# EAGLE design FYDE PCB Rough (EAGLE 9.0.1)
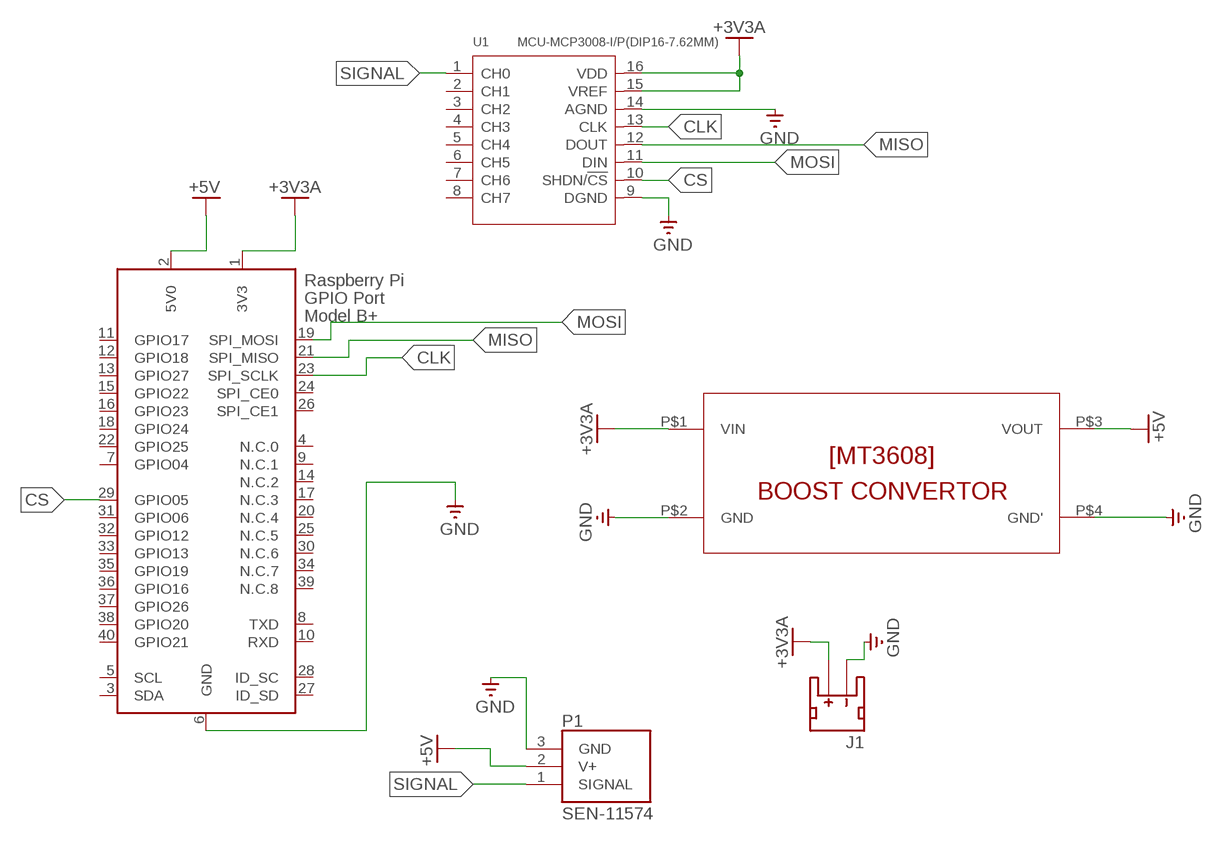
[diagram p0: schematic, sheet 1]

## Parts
J1  JST_2MM_MALE  [JST-2-SMD]
P1  SEN-11574  [XDCR_SEN-11574]
U1  MCU-MCP3008-I/P(DIP16-7.62MM)  [DIP16-2.54-19.2X7.62MM]
U$2  MT3608  [MT3608]
X1  RASPI_BOARD_B+_HDC  [RASPI_BOARD_B+HAT_DF_CF]

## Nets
+3V3A: J1.2(+) U1.15(VREF) U1.16(VDD) U$2.P$1(VIN) X1.1(3V3)
+5V: P1.2(V+) U$2.P$3(VOUT) X1.2(5V0)
CLK: U1.13(CLK) X1.23(SPI_SCLK)
CS: U1.10(SHDN/!CS) X1.29(GPIO05)
GND: J1.1(-) P1.3(GND) U1.9(DGND) U1.14(AGND) U$2.P$2(GND) U$2.P$4(GND') X1.6(GND)
MISO: U1.12(DOUT) X1.21(SPI_MISO)
MOSI: U1.11(DIN) X1.19(SPI_MOSI)
SIGNAL: P1.1(SIGNAL) U1.1(CH0)
Unconnected: J1.NC1(PAD1) J1.NC2(PAD2) U1.2(CH1) U1.3(CH2) U1.4(CH3) U1.5(CH4) U1.6(CH5) U1.7(CH6) U1.8(CH7) X1.3(SDA) X1.4(N.C.0) X1.5(SCL) X1.7(GPIO04) X1.8(TXD) X1.9(N.C.1) X1.10(RXD) X1.11(GPIO17) X1.12(GPIO18) X1.13(GPIO27) X1.14(N.C.2) X1.15(GPIO22) X1.16(GPIO23) X1.17(N.C.3) X1.18(GPIO24) X1.20(N.C.4) X1.22(GPIO25) X1.24(SPI_CE0) X1.25(N.C.5) X1.26(SPI_CE1) X1.27(ID_SD) X1.28(ID_SC) X1.30(N.C.6) X1.31(GPIO06) X1.32(GPIO12) X1.33(GPIO13) X1.34(N.C.7) X1.35(GPIO19) X1.36(GPIO16) X1.37(GPIO26) X1.38(GPIO20) X1.39(N.C.8) X1.40(GPIO21)

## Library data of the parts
J1 = SparkFun-Connectors:JST_2MM_MALE: JST 2MM MALE RA CONNECTOR Two pin, compact surface mount connector. Commonly used as a battery input connection point. We really like the solid locking feeling and high current rating on these small connectors. We use these all the time as battery connectors. Mates to single-cell LiPo batteries.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; PROD_ID: CONN-11443; SF_ID: PRT-08612
P1 = SEN-11574:SEN-11574: Pulse Sensor For Arduino; AVAILABILITY: Unavailable; DESCRIPTION: PULSE SENSOR FOR ARDUINO; MF: SparkFun; MP: SEN-11574; PACKAGE: None; PRICE: None
U1 = MCU-MCP3008-I_P_DIP16-7.62MM_:MCU-MCP3008-I/P(DIP16-7.62MM): 310990040; AVAILABILITY: Unavailable; DESCRIPTION: 10 Bit Analog to Digital Converter 4, 8 Input 1 SAR 16-PDIP; MF: Microchip; MP: MCP3008-I/P; PACKAGE: DIP-16 Microchip; PRICE: None
U$2 = MT3608:MT3608
X1 = raspberrypi_bastelstube_v13:RASPI_BOARD_B+: Raspberry Pi GPIO connector with markings for the outer dimensions of the Raspberry Pi board model B+ with different sets of drill holes or mounting pads

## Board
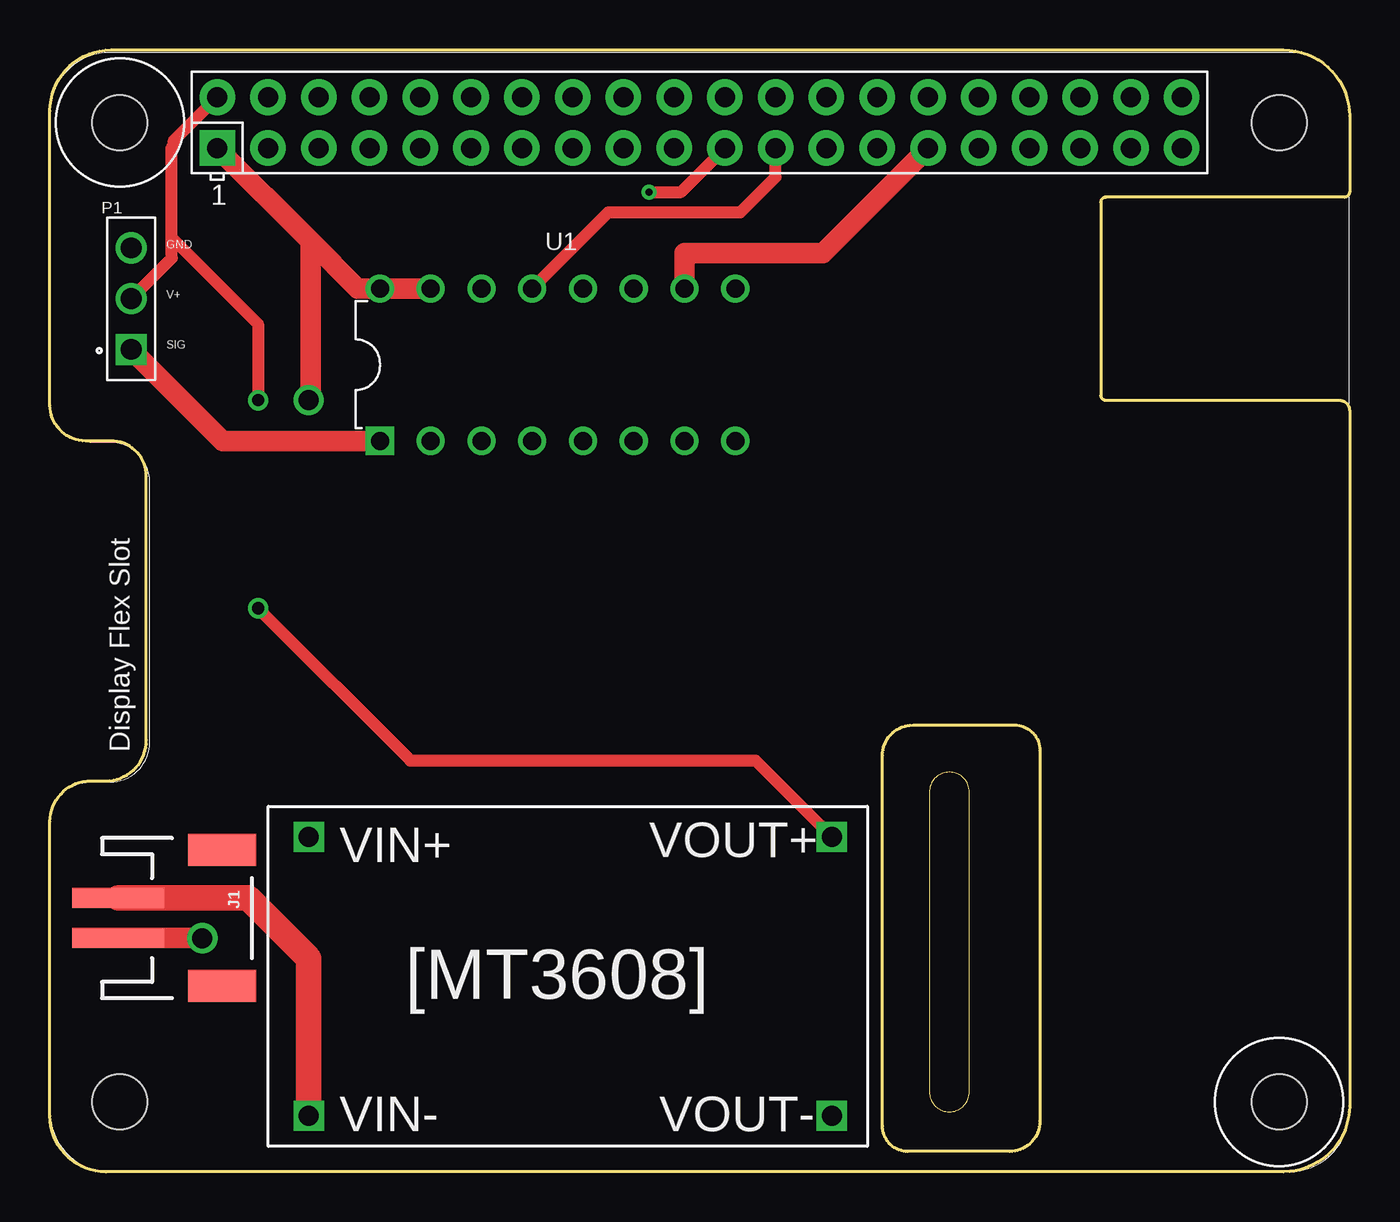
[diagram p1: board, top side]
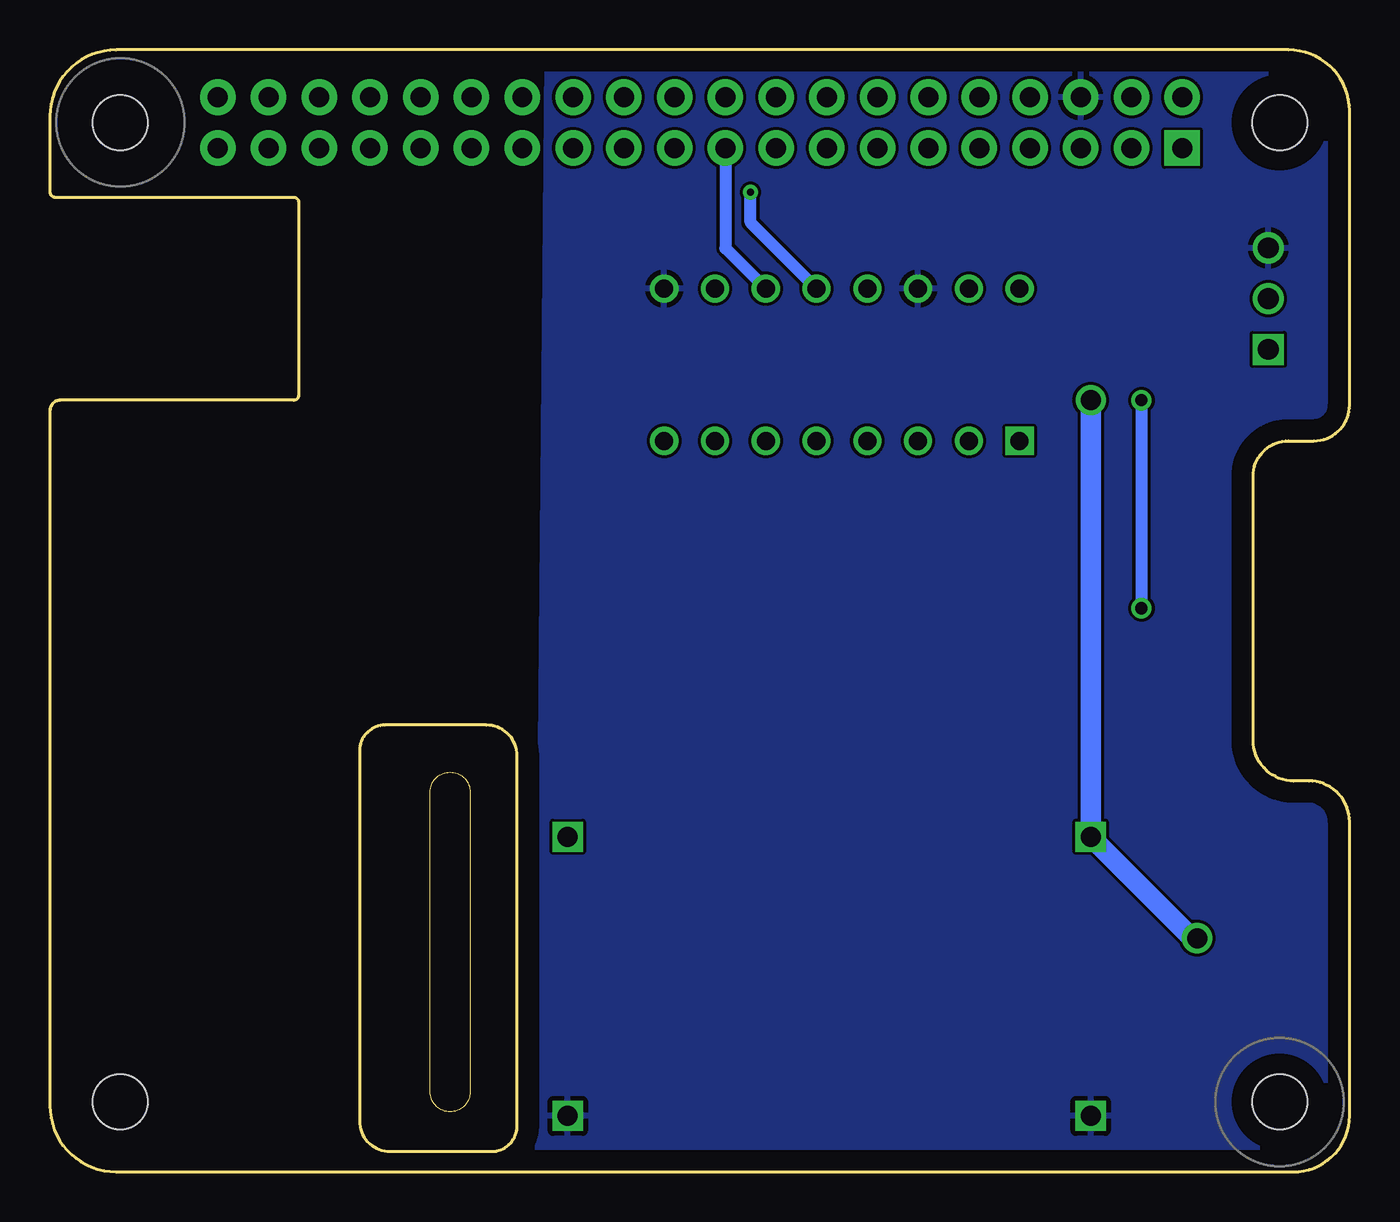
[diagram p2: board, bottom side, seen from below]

Size 65.02 x 56.13 mm. Coordinates in mm from the lower left corner, seen from the top.
Outline: 0,53.09 arc-90 3.05,56.13 61.72,56.13 arc-90 65.02,52.83 65.02,49.02 arc-90 64.77,48.77 52.83,48.77 arc90 52.58,48.51 52.58,38.86 arc90 52.83,38.61 64.52,38.61 arc-90 65.02,38.1 65.02,3.3 arc-90 61.72,0 2.79,0 arc-90 0,2.79 0,17.53 arc-90 2.03,19.56 2.79,19.56 arc90 4.83,21.59 4.83,34.8 arc90 3.05,36.58 1.78,36.58 arc-90 0,38.35 0,53.09
Outline: 41.66,2.29 41.66,20.83 arc-90 43.18,22.35 48.26,22.35 arc-90 49.53,21.08 49.53,2.54 arc-90 48.01,1.02 42.93,1.02 arc-90 41.66,2.29
Copper layers (1*16): Top 0.035mm / dielectric 1.5mm / Bottom 0.035mm
Design rules "default": minimum track width 6mil, minimum drill 0.35mm, track to track 6mil, track to pad 6mil, pad to pad 6mil, via to via 6mil, smd to smd 6mil, copper to edge 40mil, drill to drill 6mil, minimum pad ring 10mil, minimum via ring 8mil, stop-mask expansion 4mil, vias tented up to drill 0mil, thermal gap 10mil

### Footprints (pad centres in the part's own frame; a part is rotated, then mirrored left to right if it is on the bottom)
JST-2-SMD = smd 1 x 4.6: 1 -1,-3.7; 2 1,-3.7 | smd 1.6 x 3.4: NC1 -3.4,1.5; NC2 3.4,1.5
XDCR_SEN-11574 = drill 1.04 square: 1 0,-2.54 | drill 1.04: 2 0,0; 3 0,2.54
DIP16-2.54-19.2X7.62MM = drill 0.9 pad 1.4 square: 1 -8.89,-3.81 | drill 0.9 pad 1.4: 2 -6.35,-3.81; 3 -3.81,-3.81; 4 -1.27,-3.81; 5 1.27,-3.81; 6 3.81,-3.81; 7 6.35,-3.81; 8 8.89,-3.81; 9 8.89,3.81; 10 6.35,3.81; 11 3.81,3.81; 12 1.27,3.81; 13 -1.27,3.81; 14 -3.81,3.81; 15 -6.35,3.81; 16 -8.89,3.81
MT3608 = drill 1 square: P$1 2.032,15.494; P$2 2.032,1.524; P$3 28.194,15.494; P$4 28.194,1.524
RASPI_BOARD_B+HAT_DF_CF = drill 1 pad 1.778 square: 1 8.37,51.23 | drill 1 pad 1.778: 2 8.37,53.77; 3 10.91,51.23; 4 10.91,53.77; 5 13.45,51.23; 6 13.45,53.77; 7 15.99,51.23; 8 15.99,53.77; 9 18.53,51.23; 10 18.53,53.77; 11 21.07,51.23; 12 21.07,53.77; 13 23.61,51.23; 14 23.61,53.77; 15 26.15,51.23; 16 26.15,53.77; 17 28.69,51.23; 18 28.69,53.77; 19 31.23,51.23; 20 31.23,53.77; 21 33.77,51.23; 22 33.77,53.77; 23 36.31,51.23; 24 36.31,53.77; 25 38.85,51.23; 26 38.85,53.77; 27 41.39,51.23; 28 41.39,53.77; 29 43.93,51.23; 30 43.93,53.77; 31 46.47,51.23; 32 46.47,53.77; 33 49.01,51.23; 34 49.01,53.77; 35 51.55,51.23; 36 51.55,53.77; 37 54.09,51.23; 38 54.09,53.77; 39 56.63,51.23; 40 56.63,53.77 | hole 2.75: 3.5,3.5; 3.5,52.5; 61.5,3.5; 61.5,52.5

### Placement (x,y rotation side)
J1  7.11,12.7 270 top
P1  4.06,43.69 0 top
U1  25.4,40.39 0 top
U$2  10.92,1.27 0 top
X1  0,0 0 top

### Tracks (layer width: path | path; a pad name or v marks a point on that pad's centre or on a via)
+3V3A  (via drill 1, 1.02)
  Top 1.016: X1.1 13.04,46.56 | 13.04,46.56 15.4,44.2 U1.16 U1.15 | 13.04,46.56 13.04,38.69 v12.95,38.61 | J1.2 7.6,11.7 v7.62,11.68
  Bottom 1.016: v12.95,38.61 U$2.P$1 7.87,11.68 v7.62,11.68
+5V  (via drill 0.61)
  Top 0.61: P1.2 6.1,45.72 6.1,46.74 | X1.2 6.2,51.6 6.2,51.38 6.1,51.28 6.1,46.74 | 6.1,46.74 10.41,42.42 v10.41,38.61 | v10.41,28.19 18.03,20.57 32.26,20.57 35.31,20.57 U$2.P$3
  Bottom 0.61: v10.41,38.61 v10.41,28.19
CLK
  Top 0.61: U1.13 27.94,48.01 34.54,48.01 36.31,49.77 X1.23
CS
  Top 1.016: X1.29 38.67,45.97 31.75,45.97 U1.10
GND
  Top 1.27: J1.1 9.92,13.7 12.95,10.67 U$2.P$2
  pour Bottom: 0.51,55.63 1.02,0 40.64,0 40.13,55.63
MISO  (via drill 0.35)
  Top 0.61: v29.97,49.02 31.56,49.02 X1.21
  Bottom 0.61: U1.12 29.97,47.5 v29.97,49.02
MOSI
  Bottom 0.61: X1.19 31.23,46.22 U1.11
SIGNAL
  Top 1.016: P1.1 8.64,36.58 U1.1

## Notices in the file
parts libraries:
supply0: Copyright (C) 2007, Bob Starr
SparkFun-Connectors: Licensing: Creative Commons ShareAlike 4.0 International - https://creativecommons.org/licenses/by-sa/4.0
